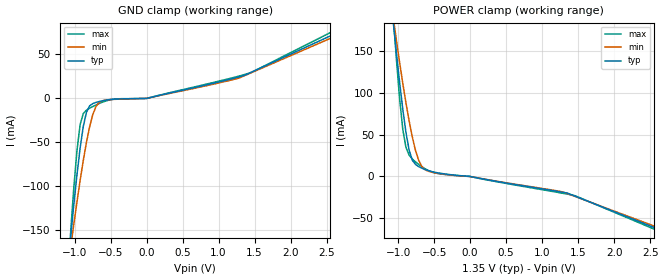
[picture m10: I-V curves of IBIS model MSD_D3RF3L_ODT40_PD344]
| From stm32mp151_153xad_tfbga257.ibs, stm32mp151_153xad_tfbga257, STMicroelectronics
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[Model] MSD_D3RF3L_ODT40_PD344
Model_type   Input
C_comp 2.270pF   2.232pF   2.321pF
Vinh = 810.000mV
Vinl = 540.000mV
[Temperature Range]   25.000   125.000   -40.000
[Voltage Range]   1.350V   1.283V   1.450V
[GND Clamp Reference]   0.00V   0.00V   0.00V
[POWER Clamp Reference]   1.350V   1.283V   1.450V
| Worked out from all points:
|   GND clamp passes 1 mA (typ) near -0.47 V on its own axis
|   POWER clamp passes 1 mA (typ) near -0.15 V on its own axis
[GND Clamp]
-1.318V   -414.9mA   -340.9mA   -532.7mA
-1.055V   -158.9mA   -170.2mA   -152.9mA
-1.011V   -121.3mA   -143.4mA   -102.2mA
-966.7mV  -86.9mA    -117.7mA   -59.43mA
-922.7mV  -56.5mA    -93.24mA   -29.85mA
-878.8mV  -31.84mA   -70.46mA   -17.23mA
-834.9mV  -15.73mA   -49.96mA   -13.3mA
-747mV    -5.846mA   -18.4mA    -9.236mA
-615.1mV  -2.742mA   -2.748mA   -4.352mA
200nV     4.014nA    3.751nA    4.249nA
1.45V     29.61mA    29.01mA    29.33mA
2.68V     75.86mA    72.8mA     80.06mA
[Power Clamp]
-1.33V    440.2mA    362.9mA    565.1mA
-1.067V   184.5mA    189.8mA    191.8mA
-1.023V   147.3mA    162.6mA    139.7mA
-978.8mV  112.5mA    136.4mA    92.94mA
-934.9mV  80.41mA    111.4mA    56.18mA
-890.9mV  52.56mA    88.03mA    34.8mA
-847mV    31.47mA    66.49mA    25.53mA
-759.1mV  14.39mA    31.35mA    17.45mA
-671.2mV  9.927mA    12.05mA    11.64mA
-583.3mV  7.051mA    6.307mA    7.248mA
1.438V    -22.96mA   -23.38mA   -22.63mA
2.668V    -65.02mA   -63.08mA   -67.24mA
